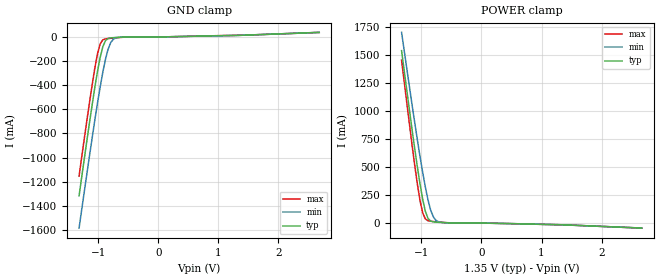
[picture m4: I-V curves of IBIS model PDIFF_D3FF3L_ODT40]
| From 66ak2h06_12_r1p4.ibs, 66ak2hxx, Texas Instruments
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|   Model PDIFF_D3FF3L_ODT40
[Model] PDIFF_D3FF3L_ODT40
Model_type   Input
Polarity   Non-Inverting
Enable   Active-High
C_comp   3.396pF   3.304pF   3.502pF
C_comp_pullup   680.121fF   623.338fF   740.323fF
C_comp_pulldown 2.710pF   2.675pF   2.755pF
Vinh = 810.000mV
Vinl = 540.000mV
[Temperature Range]   25.000   125.000   -40.000
[Voltage Range]   1.350V   1.283V   1.450V
[GND Clamp Reference]   0.00V   0.00V   0.00V
|[C Comp Corner]
| variable   typ   min   max
|C_comp 3.396pF   3.502pF   3.304pF
|C_comp_pullup 680.121fF   740.323fF   623.338fF
|C_comp_pulldown 2.710pF   2.755pF   2.675pF
[POWER Clamp Reference]   1.350V   1.283V   1.450V
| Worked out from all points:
|   GND clamp passes 1 mA (typ) near -0.59 V on its own axis
|   POWER clamp passes 1 mA (typ) near -0.49 V on its own axis
[GND Clamp]
-1.318V   -1.318A    -1.586A    -1.154A
-1.142V   -701.8mA   -977mA     -534.7mA
-1.055V   -415mA     -685.8mA   -255.7mA
-1.011V   -283.9mA   -546.7mA   -139mA
-966.7mV  -168.8mA   -414.4mA   -57.29mA
-922.7mV  -80.37mA   -292.3mA   -23.65mA
-878.8mV  -30.46mA   -185.2mA   -15.61mA
-834.9mV  -12.57mA   -100.6mA   -12.73mA
-790.9mV  -7.374mA   -45.63mA   -10.56mA
-747mV    -5.256mA   -18.36mA   -8.556mA
-571.2mV  -634.2uA   -685.4uA   -1.774mA
2.68V     38.38mA    38.18mA    37.84mA
[Power Clamp]
-1.33V    1.537A     1.7A       1.452A
-1.155V   830.5mA    1.052A     693.2mA
-1.067V   500.4mA    741.6mA    347.2mA
-1.023V   348.6mA    593.4mA    199.7mA
-978.8mV  213.2mA    452.5mA    91.09mA
-934.9mV  106.3mA    322.2mA    37.43mA
-890.9mV  42.43mA    207.9mA    20.85mA
-847mV    18.15mA    117.3mA    16.23mA
-803mV    11.17mA    56.74mA    13.69mA
-759.1mV  8.55mA     24.86mA    11.49mA
-539.4mV  1.878mA    2.107mA    2.578mA
2.668V    -44.29mA   -44.49mA   -45.17mA
